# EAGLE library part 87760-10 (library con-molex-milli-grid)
HEADER
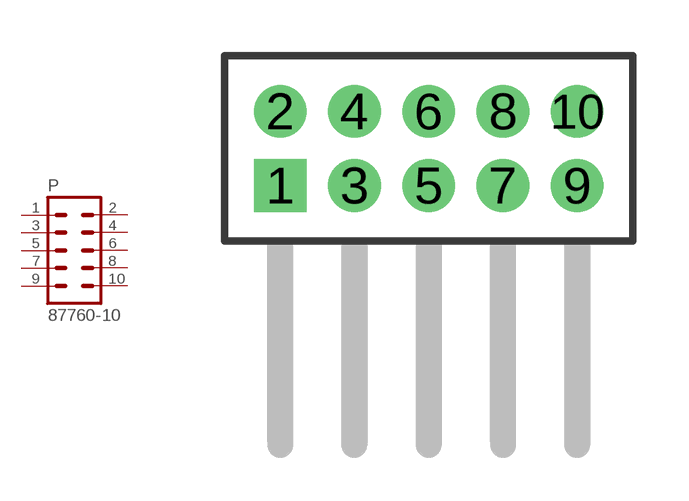
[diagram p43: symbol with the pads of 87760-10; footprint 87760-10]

Designator prefix P

## 87760-10  [87760-10]
1  1  pas
2  2  pas
3  3  pas
4  4  pas
5  5  pas
6  6  pas
7  7  pas
8  8  pas
9  9  pas
10  10  pas

## Footprint 87760-10 (pad centres in mm)
HEADER Dual Row, Right Angle
drill 0.914 square: 1 -4,-1
drill 0.914: 2 -4,1; 3 -2,-1; 4 -2,1; 5 0,-1; 6 0,1; 7 2,-1; 8 2,1; 9 4,-1; 10 4,1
